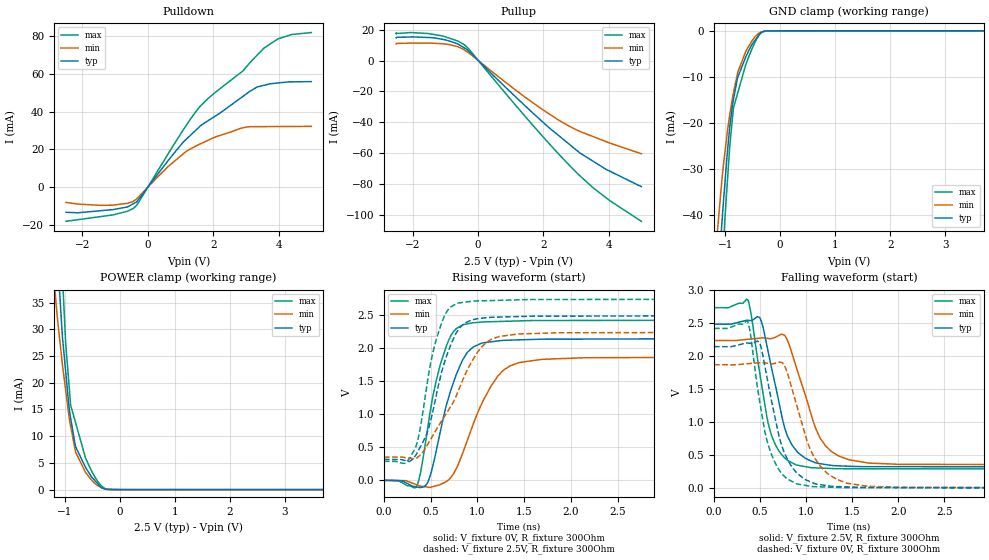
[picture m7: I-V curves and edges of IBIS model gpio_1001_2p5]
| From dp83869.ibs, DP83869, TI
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|   gpio_1001_2p5 Model
[Model]   gpio_1001_2p5
Model_type   I/O
Polarity   Non-Inverting
Enable   Active-Low
Vinl = 0.7
Vinh = 1.7
Vmeas = 1.25
Vref = 0
Cref = 2pF
Rref = 100000
|   typ   min   max
C_comp   1.246pF   1.092pF   1.323pF
| Where Nom  PVT is Nominal Process, 2.5V,  27C
|   Fast PVT is Strong Process,  2.75V, -40C
|   Slow PVT is Weak Process,   2.25V, 125C
[Voltage Range]   2.5   2.25   2.75
|Junction Temperature
[Temperature Range]   27   125   -40
[Pullup Reference]   2.5   2.25   2.75
[Pulldown Reference]   0   0   -0
[Power Clamp Reference]   2.5   2.25   2.75
[GND Clamp Reference]   0   0   0
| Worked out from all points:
|   slope of the pulldown table from 0 to 0.375 V, typ, clamps not added: 43.7 ohm
|   slope of the pullup table from 0 to 0.375 V, typ, clamps not added: 47.8 ohm
|   GND clamp passes 1 mA (typ) near -0.39 V on its own axis
|   POWER clamp passes 1 mA (typ) near -0.39 V on its own axis
|   falling waveform, V_fixture 2.5V, R_fixture 300Ohm: 20-80 % time 220ps typ, 279ps min, 187ps max; typ from 2.49 V to 0.318 V
|   rising waveform, V_fixture 0V, R_fixture 300Ohm: 20-80 % time 252ps typ, 347ps min, 211ps max; typ from 0 V to 2.14 V
|   rising waveform, V_fixture 2.5V, R_fixture 300Ohm: 20-80 % time 247ps typ, 423ps min, 200ps max; typ from 0.318 V to 2.49 V
|   falling waveform, V_fixture 0V, R_fixture 300Ohm: 20-80 % time 229ps typ, 284ps min, 199ps max; typ from 2.15 V to 0 V
[Pulldown]
|   Voltage   I(typ)   I(min)   I(max)
-2.5V     -13.28mA   -8.043mA   -18.05mA
-1.426V   -12.43mA   -9.611mA   -15.52mA
-624.7mV  -10.46mA   -8.55mA    -12.75mA
-439.4mV  -8.729mA   -7.384mA   -11.21mA
-312.7mV  -7.112mA   -5.683mA   -8.895mA
633.6mV   14.33mA    11.14mA    18.01mA
1.151V    24.99mA    18.67mA    32.09mA
1.615V    32.6mA     23.02mA    43.14mA
2.834V    47.16mA    31.16mA    60.57mA
3.343V    53.08mA    32.08mA    69.92mA
3.981V    55.23mA    32.14mA    78.56mA
5V        55.94mA    32.23mA    81.92mA
[GND Clamp]
|   Voltage   I(typ)   I(min)   I(max)
-2.5V     -325.5mA   -278mA     -374.2mA
-1.151V   -58.23mA   -45.14mA   -72.47mA
-1.062V   -42.41mA   -32.96mA   -53.36mA
-1.027V   -36.66mA   -28.83mA   -45.97mA
-1.002V   -32.9mA    -26.28mA   -40.58mA
-914.7mV  -20.9mA    -18.16mA   -24.96mA
-847.4mV  -14.87mA   -13.49mA   -16.7mA
-770.2mV  -10.08mA   -9.023mA   -13.46mA
-624.7mV  -5.69mA    -4.486mA   -7.361mA
-461.2mV  -2.152mA   -1.397mA   -2.589mA
-358.7mV  -493.6uA   -330.5uA   -623.8uA
5V        0A         0A         0A
[Pullup]
|   Voltage   I(typ)   I(min)   I(max)
-2.5V     14.74mA    10.84mA    17.55mA
-2.061V   15.36mA    11.35mA    18.2mA
-1.324V   14.72mA    11.27mA    16.85mA
-909mV    12.97mA    10.55mA    14.84mA
-438.7mV  8.572mA    7.246mA    10.61mA
-284.2mV  6.185mA    5.06mA     7.658mA
1.555V    -31.52mA   -25.4mA    -38.86mA
2.425V    -47.83mA   -37.99mA   -59.53mA
2.888V    -55.86mA   -43.57mA   -69.85mA
3.535V    -65.41mA   -49.36mA   -82.66mA
4.025V    -71.61mA   -53.4mA    -90.69mA
5V        -81.74mA   -60.39mA   -104.2mA
[POWER Clamp]
|   Voltage   I(typ)   I(min)   I(max)
-2.5V     383.1mA    300.3mA    465.8mA
-1.266V   71.49mA    49.29mA    97.35mA
-1.162V   48.95mA    35.07mA    69.59mA
-1.083V   35.09mA    27.16mA    48.6mA
-1.045V   28.71mA    23.46mA    40.28mA
-931.5mV  16.22mA    14.27mA    20.57mA
-895.2mV  13.43mA    11.92mA    15.85mA
-802.5mV  7.998mA    6.976mA    12.45mA
-624.7mV  4.17mA     3.233mA    5.928mA
-449.2mV  1.632mA    1.121mA    2.271mA
-321.9mV  342.6uA    265.3uA    574.7uA
5V        0A         0A         0A
[Ramp]
R_load = 300
|   typ   min   max
dV/dt_r   1.28602/2.50681e-10   1.11962/3.45082e-10   1.45314/2.09601e-10
dV/dt_f   1.3025/2.19414e-10   1.13234/2.78006e-10   1.47051/1.87059e-10
[Falling Waveform]
V_fixture = 2.5V
V_fixture_min = 2.25V
V_fixture_max = 2.75V
R_fixture = 300Ohm
C_fixture = 0F
|   Time   V(typ)   V(min)   V(max)
0s        2.488V     2.239V     2.737V
367.7ps   2.545V     2.257V     2.852V
498.9ps   2.579V     2.275V     1.721V
585.1ps   2.085V     2.27V      999.7mV
636.2ps   1.747V     2.273V     753.1mV
766.5ps   915.7mV    2.317V     456.5mV
889.9ps   572.9mV    1.848V     350.3mV
1.153ns   367.1mV    756.2mV    300.8mV
1.471ns   328.7mV    425.5mV    290.9mV
5ns       317.6mV    351.7mV    286.6mV
[Rising Waveform]
V_fixture = 0V
V_fixture_min = 0V
V_fixture_max = 0V
R_fixture = 300Ohm
C_fixture = 0F
|   Time   V(typ)   V(min)   V(max)
0s        128.6uV    227.6uV    124.8uV
352.6ps   -101.3mV   -68.89mV   -84.03mV
395.7ps   -108.4mV   -88.03mV   145.9mV
466.7ps   -37.27mV   -102.4mV   774.4mV
599.5ps   709mV      -66.24mV   1.729V
719ps     1.376V     50.71mV    2.193V
847.2ps   1.831V     426.6mV    2.35V
1.158ns   2.094V     1.449V     2.397V
1.453ns   2.122V     1.781V     2.409V
5ns       2.143V     1.866V     2.422V
[Rising Waveform]
V_fixture = 2.5V
V_fixture_min = 2.25V
V_fixture_max = 2.75V
R_fixture = 300Ohm
C_fixture = 0F
|   Time   V(typ)   V(min)   V(max)
0s        317.6mV    351.7mV    286.6mV
228.8ps   298mV      343.6mV    257.6mV
334.8ps   368.6mV    325.4mV    484.2mV
456.8ps   695.7mV    515.2mV    1.409V
560.1ps   1.282V     763.6mV    2.129V
665.3ps   1.858V     1.005V     2.532V
782.5ps   2.244V     1.306V     2.674V
1.003ns   2.441V     1.937V     2.71V
1.235ns   2.466V     2.173V     2.719V
5ns       2.488V     2.239V     2.737V
[Falling Waveform]
|Gnd
V_fixture = 0V
V_fixture_min = 0V
V_fixture_max = 0V
R_fixture = 300Ohm
C_fixture = 0F
|   Time   V(typ)   V(min)   V(max)
0s        2.146V     1.871V     2.423V
365.2ps   2.2V       1.886V     2.524V
489.1ps   2.216V     1.9V       1.366V
569.2ps   1.721V     1.895V     749.2mV
651.4ps   1.141V     1.889V     415.5mV
757.6ps   553mV      1.873V     181.8mV
889.9ps   240.1mV    1.295V     64.71mV
1.089ns   66.06mV    461.1mV    18.62mV
1.453ns   13.66mV    68.24mV    4.224mV
5ns       127.1uV    224.9uV    124.4uV
